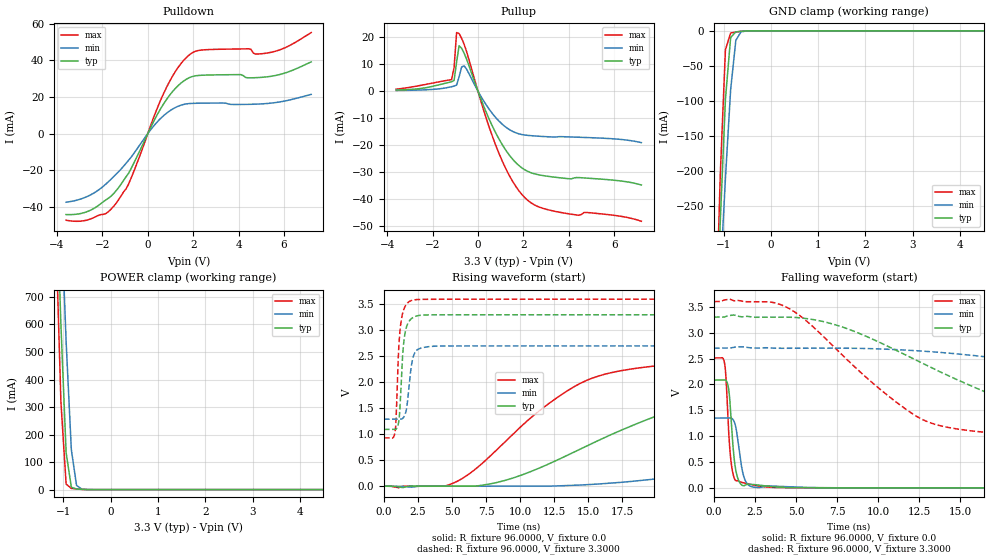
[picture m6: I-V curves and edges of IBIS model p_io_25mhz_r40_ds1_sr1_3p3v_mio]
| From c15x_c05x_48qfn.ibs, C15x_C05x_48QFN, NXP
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[Model] p_io_25mhz_r40_ds1_sr1_3p3v_mio
|   Model p_io_25mhz_r40_ds1_sr1_3p3v_mio
| This model was characterised for following simulation conditions:
| External (pad) voltage:
|   - Typ: 3.3V,   - Min: 2.7V,   - Max: 3.6V
| Library cells for typ/min/max conditions are connected as defined below:
|  pad - External Pad
|  ipp_do_lv - Core Input
|  ipp_obe_lv - Output Buffer Enable
|  IOGC - NC
|  REFH3V3 - REFH3V3
|  REFL3V3 - REFL3V3
|  ZI - NC
|  abut_ncal_vddio[1] - vddio
|  abut_ncal_vddio[2] - vddio
|  abut_ncal_vddio[3] - vssio
|  abut_ncal_vddio[4] - vddio
|  abut_ncal_vddio[5] - vddio
|  abut_ncal_vddio[6] - vssio
|  abut_pcal_vddio[1] - vssio
|  abut_pcal_vddio[2] - vssio
|  abut_pcal_vddio[3] - vddio
|  abut_pcal_vddio[4] - vssio
|  abut_pcal_vddio[5] - vssio
|  abut_pcal_vddio[6] - vddio
|  ipp_do_1p8v - ipp_do_1p8v
|  ipp_dse_lv - vdd_lv
|  ipp_eftd_lv - NC
|  ipp_ina_mux_vddio - NC
|  ipp_ina_mux_vddio[0] - NC
|  ipp_ina_mux_vddio[1] - NC
|  ipp_ina_r0_vddio - NC
|  ipp_ina_r0a_vddio - NC
|  ipp_ina_r0b_vddio - NC
|  ipp_ina_r0c_vddio - NC
|  ipp_ina_r0d_vddio - NC
|  ipp_ina_r0e_vddio - NC
|  ipp_ina_r0f_vddio - NC
|  ipp_ina_r300_vddio - NC
|  ipp_ina_r300a_vddio - NC
|  ipp_ina_r300b_vddio - NC
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Model_type I/O
Polarity   Non-Inverting
Enable   Active-High
Vinl =   0.9900V
Vinh =   2.3100V
Vmeas =  1.6500V
Cref =   30.0000pF
Rref =   1.0000M
Vref =   3.3000V
C_comp   1.6860pF   1.6265pF   1.7672pF
|C_comp_pullup   0.5958pF   0.6269pF   0.5746pF
|C_comp_pulldown   0.8297pF   0.8781pF   0.7921pF
[Model Spec]
| variable   typ   min   max
Vinh   2.3100V   1.8900V   2.5200V
Vinl   0.9900V   0.8100V   1.0800V
[Temperature Range]   25.0000   0.1250k   -40.0000
[Voltage Range]   3.3000V   2.7000V   3.6000V
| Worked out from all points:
|   slope of the pulldown table from 0 to 0.495 V, typ, clamps not added: 40.9 ohm
|   slope of the pullup table from 0 to 0.495 V, typ, clamps not added: 47.8 ohm
|   GND clamp passes 1 mA (typ) near -0.67 V on its own axis
|   POWER clamp passes 1 mA (typ) near -0.62 V on its own axis
|   rising waveform, R_fixture 96.0000, V_fixture 0.0: 20-80 % time 12ns typ, 25.6ns min, 7.17ns max; typ from 0 V to 2.08 V
|   rising waveform, R_fixture 96.0000, V_fixture 3.3000: 20-80 % time 316ps typ, 382ps min, 290ps max; typ from 1.09 V to 3.3 V
|   falling waveform, R_fixture 96.0000, V_fixture 0.0: 20-80 % time 318ps typ, 389ps min, 288ps max; typ from 2.08 V to 0 V
|   falling waveform, R_fixture 96.0000, V_fixture 3.3000: 20-80 % time 9.45ns typ, 20.5ns min, 5.74ns max; typ from 3.3 V to 1.09 V
[Pulldown]
|Voltage   I(typ)   I(min)   I(max)
-3.6V     -44.24mA   -37.49mA   -47.33mA
-2.5V     -41.72mA   -33.35mA   -46.54mA
-1.84V    -36.2mA    -27.49mA   -43.67mA
-1.4V     -31.29mA   -22.21mA   -38.12mA
-850mV    -21.76mA   -14.6mA    -27.7mA
800mV     18.19mA    10.89mA    24.63mA
1.35V     26.39mA    15.02mA    36.42mA
1.9V      30.94mA    16.48mA    43.69mA
4.43V     30.49mA    15.99mA    46.36mA
4.76V     30.57mA    16.1mA     43.49mA
5.31V     31.12mA    16.52mA    44.14mA
7.2V      39.23mA    21.44mA    55.22mA
[Pullup]
|Voltage   I(typ)   I(min)   I(max)
-3.6V     375.6uA    207.3uA    723.2uA
-1.16V    3.421mA    1.609mA    4.222mA
-1.05V    3.932mA    1.826mA    8.69mA
-940mV    10.66mA    2.21mA     21.59mA
-830mV    16.71mA    5.23mA     21.25mA
-720mV    15.83mA    8.864mA    19.49mA
-610mV    14.01mA    9.303mA    17.31mA
820mV     -16.02mA   -10.13mA   -20.77mA
1.48V     -24.67mA   -14.68mA   -32.64mA
2.03V     -28.89mA   -16.19mA   -39.05mA
3.35V     -31.77mA   -16.98mA   -44.33mA
7.2V      -34.69mA   -19.04mA   -48.08mA
[GND_clamp]
|Voltage   I(typ)   I(min)   I(max)
-3.6V     -5.343A    -4.159A    -6.913A
-1.18V    -470.5mA   -501mA     -462.9mA
-1.07V    -274.4mA   -353mA     -207.6mA
-960mV    -98.09mA   -211.4mA   -27.2mA
-850mV    -9.59mA    -84.32mA   -3.159mA
-740mV    -1.542mA   -13.52mA   -1.688mA
-630mV    -656uA     -1.44mA    -722.1uA
-300mV    -859.4nA   -5.611uA   -163.9nA
7.2V      0A         0A         0A
[POWER_clamp]
|Voltage   I(typ)   I(min)   I(max)
-3.6V     14.48A     12.95A     16.35A
-1.16V    1.177A     1.535A     951.2mA
-1.05V    598.4mA    1.032A     318mA
-940mV    134.2mA    537.3mA    20.05mA
-830mV    8.719mA    145.4mA    4.267mA
-720mV    2.135mA    15.38mA    2.236mA
-610mV    852.8uA    1.854mA    844.7uA
7.2V      0A         0A         0A
[Ramp]
| variable   typ   min   max
dV/dt_r  1.2494/12.0352n   0.8026/25.5541n   1.5064/7.1707n
dV/dt_f  1.3244/9.4531n   0.8432/20.4513n   1.6019/5.7398n
R_load = 96.0000
[Rising Waveform]
R_fixture= 96.0000
V_fixture= 0.0
V_fixture_min= 0.0
V_fixture_max= 0.0
|time   V(typ)   V(min)   V(max)
0s        3.106nV    104.7nV    10.55nV
4.705ns   -77.72uV   -323.7uV   21.01mV
8.635ns   92.71mV    7.052uV    788.9mV
11.63ns   373.4mV    601.3uV    1.495V
14.79ns   759.8mV    27.25mV    2.025V
21.4ns    1.479V     182.8mV    2.349V
31.51ns   1.889V     547.5mV    2.459V
43.65ns   2.007V     954.4mV    2.494V
54.98ns   2.048V     1.14V      2.505V
127.4ns   2.082V     1.338V     2.511V
[Rising Waveform]
R_fixture= 96.0000
V_fixture= 3.3000
V_fixture_min= 2.7000
V_fixture_max= 3.6000
|time   V(typ)   V(min)   V(max)
0s        1.093V     1.289V     930.2mV
819.7ps   1.091V     1.289V     1.048V
894ps     1.101V     1.289V     1.311V
1.117ns   1.302V     1.289V     2.792V
1.367ns   2.495V     1.302V     3.323V
1.502ns   2.867V     1.35V      3.433V
1.68ns    3.083V     1.526V     3.512V
2.053ns   3.232V     2.373V     3.576V
2.431ns   3.278V     2.621V     3.592V
127.4ns   3.3V       2.7V       3.6V
[Falling Waveform]
R_fixture= 96.0000
V_fixture= 0.0
V_fixture_min= 0.0
V_fixture_max= 0.0
|time   V(typ)   V(min)   V(max)
0s        2.083V     1.349V     2.511V
642.1ps   2.085V     1.349V     2.404V
726.5ps   2.076V     1.349V     2.126V
841.9ps   1.99V      1.349V     1.369V
970.9ps   1.647V     1.351V     706.6mV
1.248ns   499.8mV    1.262V     171.7mV
1.514ns   131.2mV    760.9mV    125.9mV
1.942ns   59.73mV    114.4mV    86.07mV
3.356ns   28.84mV    36.29mV    12.37mV
127.4ns   225.1nV    4.513uV    23.03nV
[Falling Waveform]
R_fixture= 96.0000
V_fixture= 3.3000
V_fixture_min= 2.7000
V_fixture_max= 3.6000
|time   V(typ)   V(min)   V(max)
0s        3.3V       2.7V       3.6V
4.331ns   3.299V     2.698V     3.505V
7.553ns   3.137V     2.699V     2.647V
12.33ns   2.464V     2.651V     1.383V
17.66ns   1.708V     2.492V     1.046V
20.92ns   1.412V     2.354V     996.9mV
25.36ns   1.268V     2.146V     965mV
36.26ns   1.153V     1.67V      939.4mV
46.94ns   1.119V     1.472V     933.2mV
127.4ns   1.093V     1.295V     930.2mV
